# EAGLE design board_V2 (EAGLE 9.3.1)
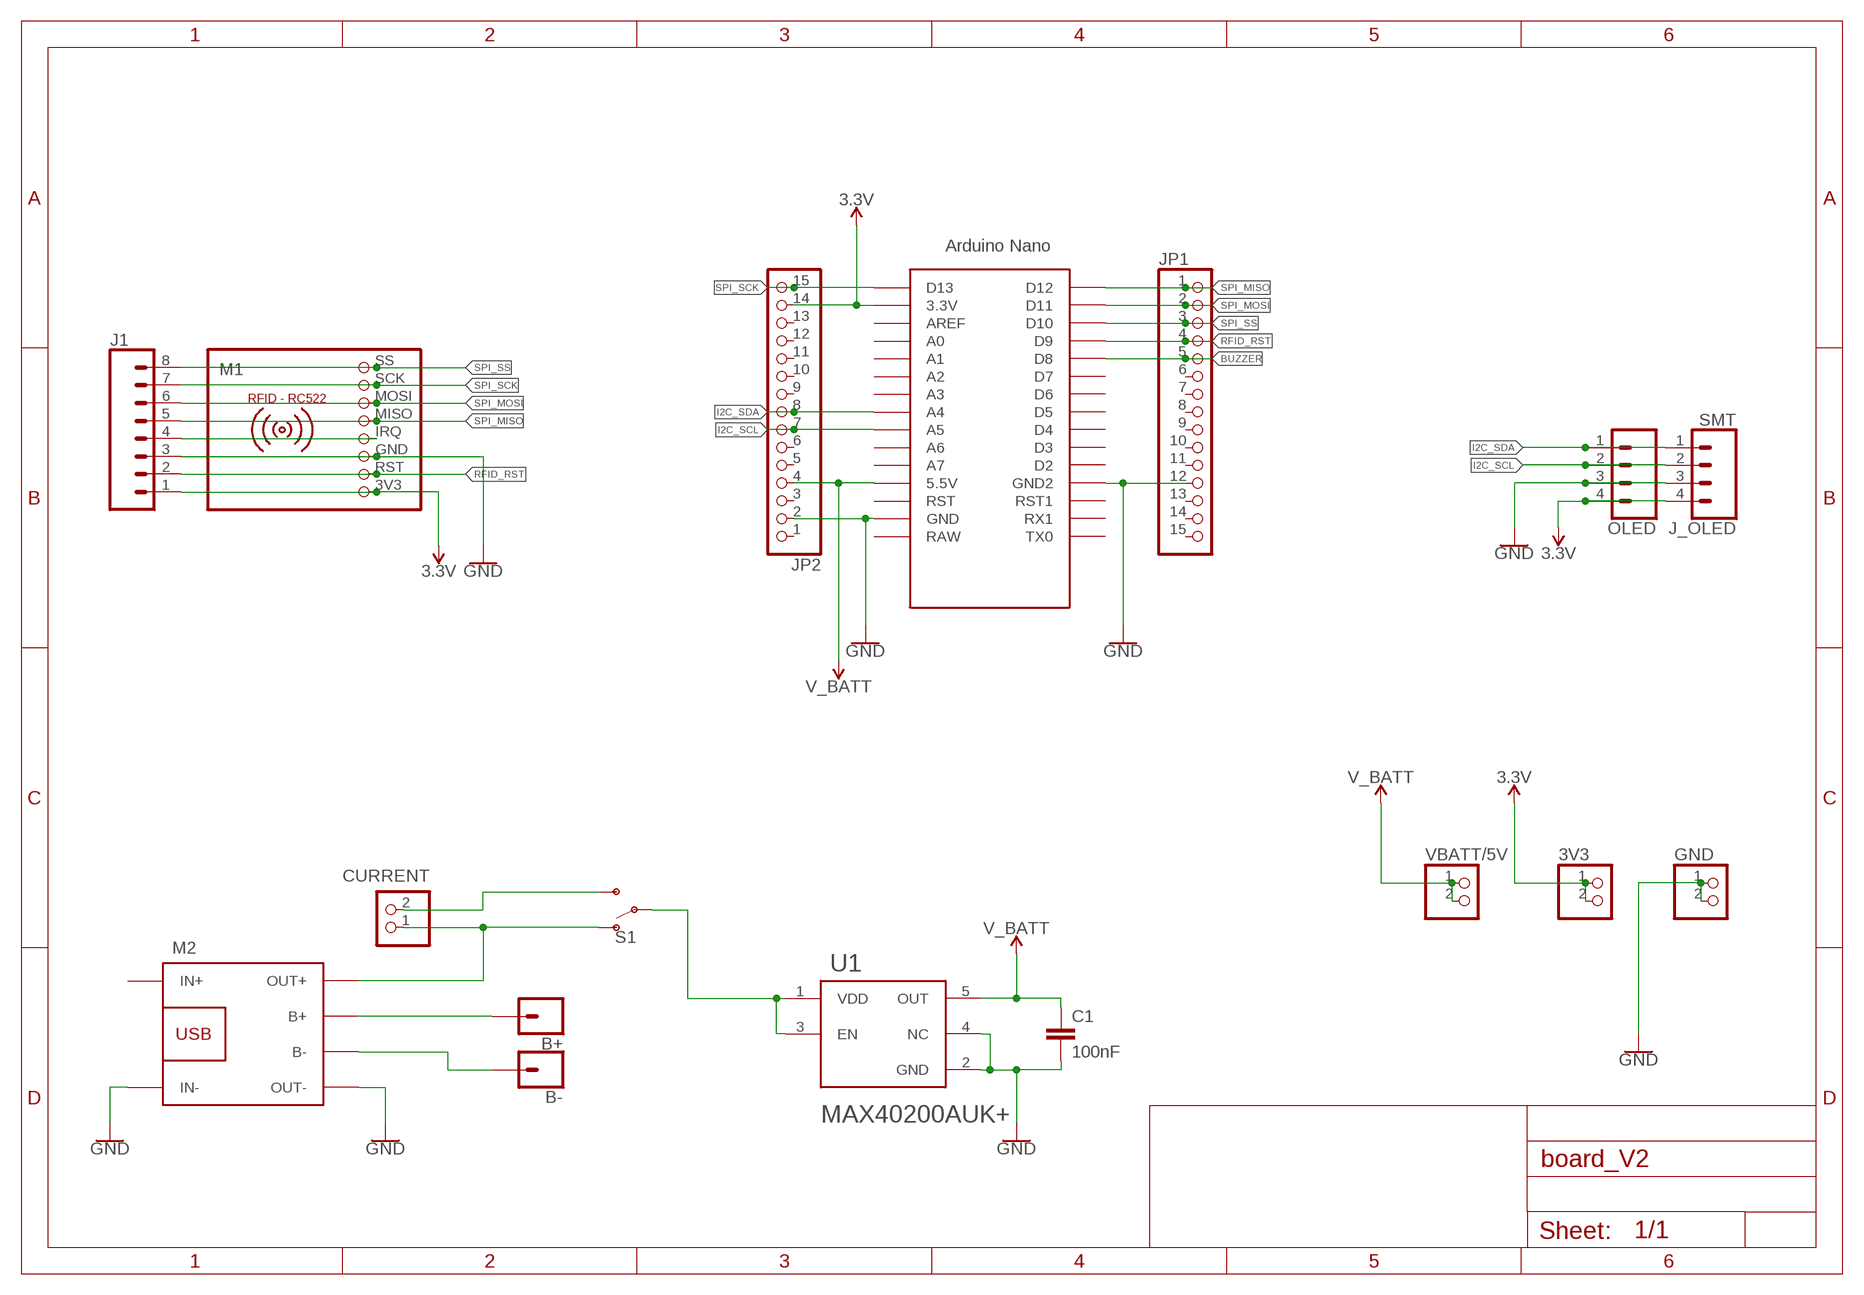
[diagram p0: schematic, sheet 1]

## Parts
3V3  PINHD-1X2  [1X02]
B+  CONN_01OFFSET  [1X01_OFFSET]
B-  CONN_01OFFSET  [1X01_OFFSET]
C1  100nF  C-EUC0805  [C0805]
CURRENT  PINHD-1X2  [1X02]
GND  PINHD-1X2  [1X02]
J1  CONN_08SMD-COMBO-FEMALE  [1X08_SMD_COMBINED]
J_OLED  SMT  CONN_04SMD_STRAIGHT_COMBO  [1X04_SMD_VERTICAL_COMBO]
JP1  PINHD-1X151X15_SMT  [1X15_SMT]
JP2  PINHD-1X151X15_SMT  [1X15_SMT]
M1  RFID-RC522  [RFID-RC522]
M2  BATTERY-CHARGER-LI-PROT  [BATTERY-CHARGER-LI-PROT]
OLED  CONN_04  [1X04]
S1  SWITCH-SPDT-PTH-11.6X4.0MM  [SWITCH_SPDT_PTH_11.6X4.0MM]
U1  MAXIM_ELECTRONICS_MAX40200AUK+MAXIM_ELECTRONICS_MAX40200AUK+_0_0  [MAXIM_ELECTRONICS_MAX40200AUK+_0]
U$1  NANO_ICSP-REMOVED  [NANO_ICSP-REMOVED]
VBATT/5V  PINHD-1X2  [1X02]

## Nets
3.3V [power]: 3V3.1 3V3.2 J1.1 J_OLED.4 JP2.14 M1.3V3 OLED.4 U$1.3.3V
BATT_VOUT [power]: S1.2(P) U1.1(VDD) U1.3(EN)
BUZZER: JP1.5 U$1.D8
GND [power]: C1.2 GND.1 GND.2 J1.3 J_OLED.3 JP1.12 JP2.2 M1.GND M2.IN- M2.OUT- OLED.3 U1.2(GND) U1.4(NC) U$1.GND U$1.GND1(GND2)
I2C_SCL: J_OLED.2 JP2.7 OLED.2 U$1.A5
I2C_SDA: J_OLED.1 JP2.8 OLED.1 U$1.A4
N$1 [power]: B+.1 M2.B+
N$2 [power]: CURRENT.1 M2.OUT+ S1.1(O)
N$3: J1.4 M1.IRQ
N$4 [power]: CURRENT.2 S1.3(S)
N$5 [power]: B-.1 M2.B-
RFID_RST: J1.2 JP1.4 M1.RST U$1.D9
SPI_MISO: J1.5 JP1.1 M1.MISO U$1.D12
SPI_MOSI: J1.6 JP1.2 M1.MOSI U$1.D11
SPI_SCK: J1.7 JP2.15 M1.SCK U$1.D13
SPI_SS: J1.8 JP1.3 M1.SS U$1.D10
V_BATT [power]: C1.1 JP2.4 U1.5(OUT) U$1.5V(5.5V) VBATT/5V.1 VBATT/5V.2
Unconnected: JP1.6 JP1.7 JP1.8 JP1.9 JP1.10 JP1.11 JP1.13 JP1.14 JP1.15 JP2.1 JP2.3 JP2.5 JP2.6 JP2.9 JP2.10 JP2.11 JP2.12 JP2.13 M2.IN+ U$1.A0 U$1.A1 U$1.A2 U$1.A3 U$1.A6 U$1.A7 U$1.AREF U$1.D2 U$1.D3 U$1.D4 U$1.D5 U$1.D6 U$1.D7 U$1.RAW U$1.RST U$1.RST1 U$1.RX1 U$1.TX0

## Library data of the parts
3V3 CURRENT GND VBATT/5V = pinhead:PINHD-1X2: PIN HEADER
B+ B- = SparkFun-Connectors:CONN_01: Single connection point. Often used as Generic Header-pin footprint for 0.1 inch spaced/style header connections
C1 = rcl:C-EU: CAPACITOR, European symbol; SPICEPREFIX: C
J1 = SparkFun-Connectors:CONN_08: Multi connection point. Often used as Generic Header-pin footprint for 0.1 inch spaced/style header connections On any of the 0.1 inch spaced packages, you can populate with these: Break Away Headers - Straight (PRT-00116) Break Away Male Headers - Right Angle (PRT-00553) Female Headers (PRT-00115)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; PROD_ID: CONN-10204; SF_ID: PRT-11543
J_OLED = SparkFun-Connectors:CONN_04: Multi connection point. Often used as Generic Header-pin footprint for 0.1 inch spaced/style header connections On any of the 0.1 inch spaced packages, you can populate with these: Break Away Headers - Straight (PRT-00116) Break Away Male Headers - Right Angle (PRT-00553) Female Headers (PRT-00115)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; PROD_ID: CONN-08511; VALUE: 1X04_SMD_STRAIGHT_COMBO
JP1 JP2 = pinhead+:PINHD-1X15: PIN HEADER
M1 = mfrc522-module:RFID-RC522: RFID-RC522 MFRC-522 based breakout board
M2 = diy-modules:BATTERY-CHARGER-LI-PROT: Lithium Battery 5V Charger with protection circuit More details available here: http://www.instructables.com/id/DIY-Lithium-ion-Battery-Charger/step4/TP4056-based-lithium-ion-battery-charger-module/ Click here to find device on ebay.com
OLED = SparkFun-Connectors:CONN_04: Multi connection point. Often used as Generic Header-pin footprint for 0.1 inch spaced/style header connections On any of the 0.1 inch spaced packages, you can populate with these: Break Away Headers - Straight (PRT-00116) Break Away Male Headers - Right Angle (PRT-00553) Female Headers (PRT-00115)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; PROD_ID: CONN-09696
S1 = SparkFun-Switches:SWITCH-SPDT: Single Pole, Double Throw (SPDT) Switch Single-pole, double-throw (SPDT) switch. Variant Overview SMD-AYZ0202 Surface Mount DPDT Switch (COM-00597) Used on e.g. LilyPad Arduino USB - ATmega32U4 Board PTH-11.6X4.0MM SPDT Mini Power Switch (COM-00102) Used on e.g. SparkFun Simon Says - Through-Hole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; PROD_ID: SWCH-08261; SF_SKU: COM-00102
U1 = Maxim Electronics - MAX40200AUK+:MAXIM_ELECTRONICS_MAX40200AUK+: IDEAL DIODE CURRENT SW, 5.5V, SOT23-5; CENTROID_NOT_SPECIFIED: No; DATASHEET: https://datasheets.maximintegrated.com/en/ds/MAX40200.pdf; DEVICE_CLASS_L1: Integrated Circuits (ICs); DEVICE_CLASS_L2: Power Management ICs; DEVICE_CLASS_L3: unset; DIGIKEY_DESCRIPTION: IC DIODE CURRENT SWITCH SOT23-5; DIGIKEY_PART_NUMBER: MAX40200AUK+-ND; FOOTPRINT_URL: https://pdfserv.maximintegrated.com/land_patterns/90-0174.PDF; HEIGHT: 1.45mm; LEAD_FREE: yes; MAX_JUNCTION_TEMP: +150°C; MAX_POWER_DISSIPATION: 312.6mW; MAX_SUPPLY_VOLTAGE: 5.5V; MF: Maxim Electronics; MFG_PACKAGE_IDENT: U5-1; MFG_PACKAGE_IDENT_DATE: 0; MFG_PACKAGE_IDENT_REV: J; MIN_SUPPLY_VOLTAGE: 1.5V; MOUSER_PART_NUMBER: 700-MAX40200AUK+; MPN: MAX40200AUK+; NOMINAL_SUPPLY_CURRENT: 7uA; NUMBER_OF_OUTPUTS: 1; OUTPUT_CURRENT: 1A; PACKAGE: SOT23-5; PREFIX: U; ROHS: yes; STANDOFF_HEIGHT: 0mm; TEMPERATURE_RANGE_HIGH: +125°C; TEMPERATURE_RANGE_LOW: -40°C; VERIFICATION_VERSION: 0.0.0.1
U$1 = Arduino-clone:NANO_ICSP-REMOVED

## Module BUZZER
Ports: 

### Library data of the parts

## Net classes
1 power: width 0.914 mm, clearance 0.254 mm

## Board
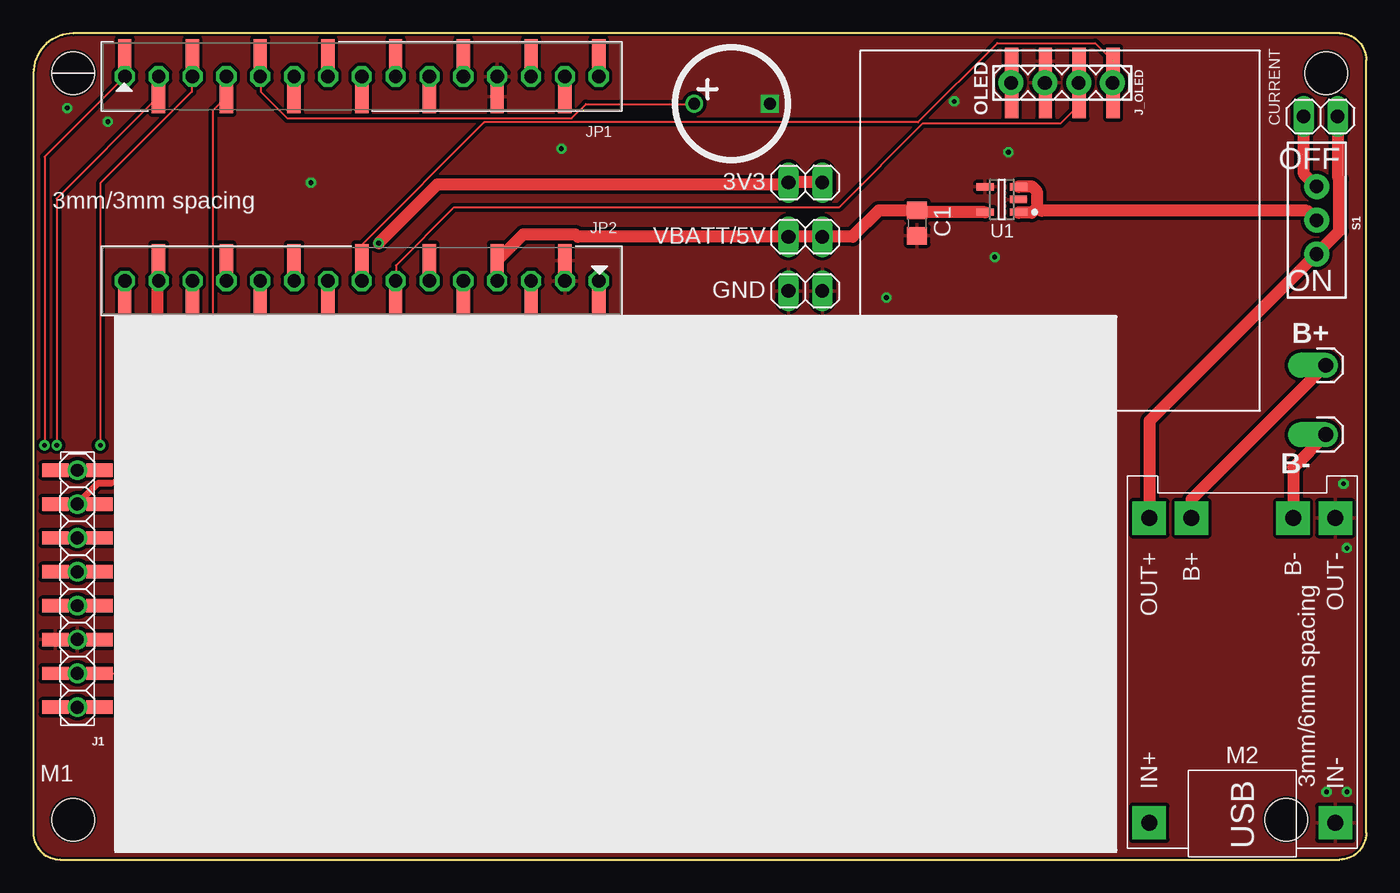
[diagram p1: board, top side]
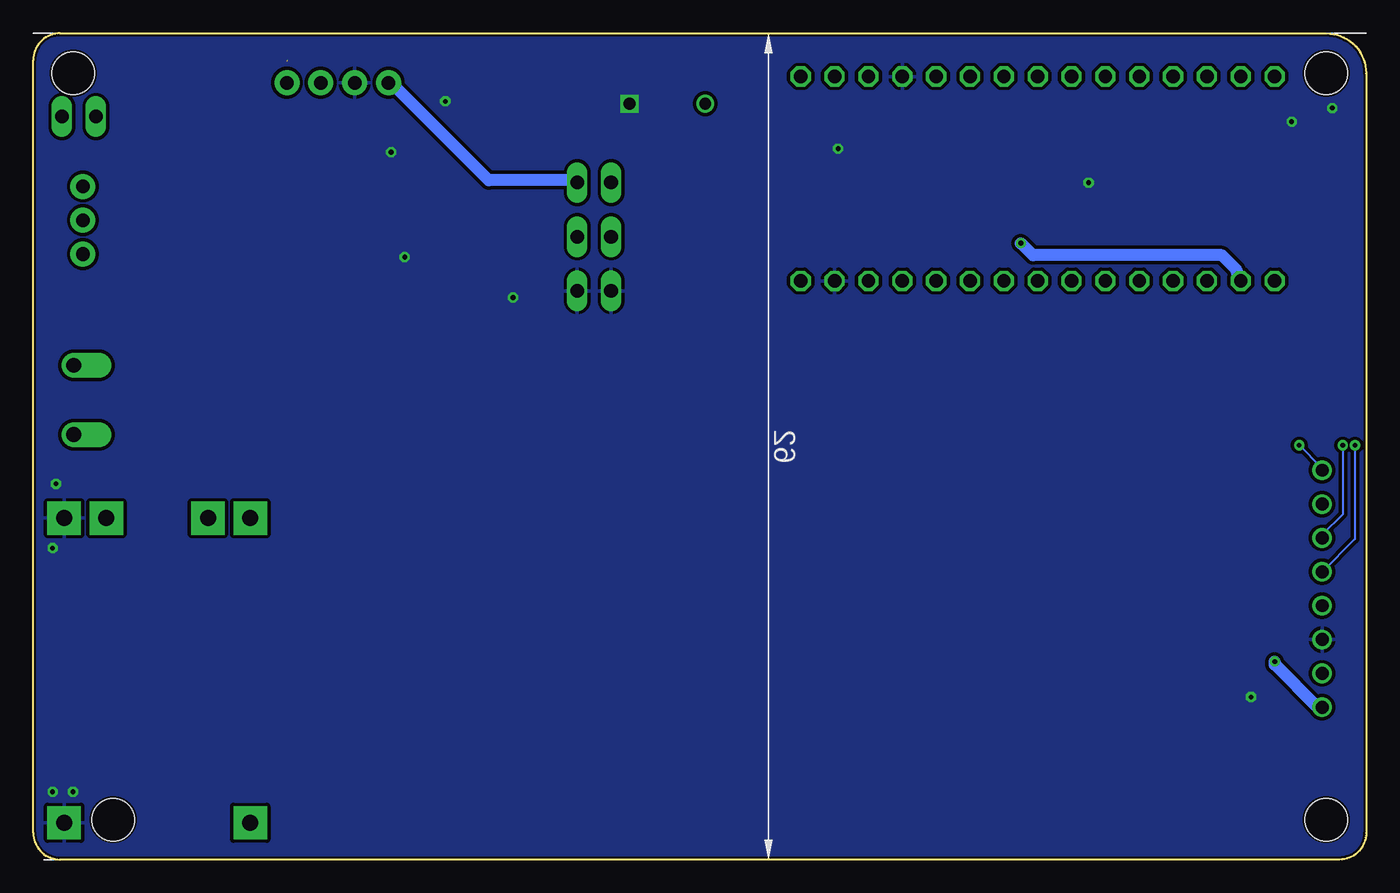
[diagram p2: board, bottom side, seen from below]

Size 100 x 62 mm. Coordinates in mm from the lower left corner, seen from the top.
Outline: 2,0 98,0 arc90 100,2 100,60 arc90 98,62 3,62 arc90 0,59 0,2 arc90 2,0
Copper layers (1*16): Top 0.035mm / dielectric 1.5mm / Bottom 0.035mm
Design rules "default *": minimum track width 6mil, minimum drill 0.35mm, track to track 6mil, track to pad 6mil, pad to pad 6mil, via to via 6mil, smd to smd 6mil, copper to edge 6mil, drill to drill 6mil, minimum pad ring 10mil, minimum via ring 8mil, stop-mask expansion 4mil, vias tented up to drill 0mil, thermal gap 10mil
Holes 3.2 mm at 3,59 3,3 94,3 97,59

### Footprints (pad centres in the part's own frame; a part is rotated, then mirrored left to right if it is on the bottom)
1X02 = drill 1.016 long: 1 -1.27,0; 2 1.27,0
1X01_OFFSET = drill 1.118 pad 1.88 offset: 1 0,0
C0805 = smd 1.3 x 1.5: 1 -0.95,0; 2 0.95,0
1X08_SMD_COMBINED = smd 1 x 2: 1 0,1.65; 1@2 0,-1.65; 2 2.54,-1.65; 2@2 2.54,1.65; 3 5.08,1.65; 3@2 5.08,-1.65; 4 7.62,-1.65; 4@2 7.62,1.65; 5 10.16,1.65; 5@2 10.16,-1.65; 6 12.7,-1.65; 6@2 12.7,1.65; 7 15.24,1.65; 7@2 15.24,-1.65; 8 17.78,-1.65; 8@2 17.78,1.65
1X04_SMD_VERTICAL_COMBO = smd 1 x 2: 1 0,-1.65; 1-2 0,1.65; 2 2.54,1.65; 2-2 2.54,-1.65; 3 5.08,-1.65; 3-2 5.08,1.65; 4 7.62,1.65; 4-2 7.62,-1.65
1X15_SMT = smd 1 x 2.5: 1 -17.78,1.52; 2 -15.24,-1.52; 3 -12.7,1.52; 4 -10.16,-1.52; 5 -7.62,1.52; 6 -5.08,-1.52; 7 -2.54,1.52; 8 0,-1.52; 9 2.54,1.52; 10 5.08,-1.52; 11 7.62,1.52; 12 10.16,-1.52; 13 12.7,1.52; 14 15.24,-1.52; 15 17.78,1.52
RFID-RC522 = drill 0.965: 3V3 -8.89,0; GND -3.81,0; IRQ -1.27,0; MISO 1.27,0; MOSI 3.81,0; RST -6.35,0; SCK 6.35,0; SS 8.89,0
BATTERY-CHARGER-LI-PROT = drill 1.2 pad 2.5 square: B+ 10.795,3.81; B- 10.795,-3.81; IN+ -12.065,6.985; IN- -12.065,-6.985; OUT+ 10.795,6.985; OUT- 10.795,-6.985
1X04 = drill 1.016 pad 1.88: 1 0,0; 2 2.54,0; 3 5.08,0; 4 7.62,0
SWITCH_SPDT_PTH_11.6X4.0MM = drill 1.016 pad 1.88: 1 0,2.54; 2 0,0; 3 0,-2.54
MAXIM_ELECTRONICS_MAX40200AUK+_0 = smd 1.3 x 0.55: 1 -1.25,0.95; 2 -1.25,0; 3 -1.25,-0.95; 4 1.25,-0.95; 5 1.25,0.95
NANO_ICSP-REMOVED = drill 1 octagon: 3.3V -10.16,24.13; 5V -10.16,-1.27; A0 -10.16,19.05; A1 -10.16,16.51; A2 -10.16,13.97; A3 -10.16,11.43; A4 -10.16,8.89; A5 -10.16,6.35; A6 -10.16,3.81; A7 -10.16,1.27; AREF -10.16,21.59; D2 5.182,1.27; D3 5.182,3.81; D4 5.182,6.35; D5 5.182,8.89; D6 5.182,11.43; D7 5.182,13.97; D8 5.182,16.51; D9 5.182,19.05; D10 5.182,21.59; D11 5.182,24.13; D12 5.182,26.67; D13 -10.16,26.67; GND -10.16,-6.35; GND1 5.182,-1.27; RAW -10.16,-8.89; RST -10.16,-3.81; RST1 5.182,-3.81; RX1 5.182,-6.35; TX0 5.182,-8.89

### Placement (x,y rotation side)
3V3  57.93,50.8 180 top
B+  96.96,37.09 90 top
B-  96.96,31.88 90 top
C1  66.31,47.75 270 top
CURRENT  96.58,55.75 180 top
GND  57.93,42.67 180 top
J1  3.3,11.43 90 top
J_OLED  81.01,58.27 180 top
JP1  24.64,58.77 0 top
JP2  24.64,43.43 180 top
M1  3.3,20.32 90 top
M2  90.7,14.82 90 top
OLED  80.97,58.29 180 top
S1  96.28,47.97 180 top
U1  72.66,49.53 180 top
U$1  33.53,53.58 90 top
VBATT/5V  57.93,46.74 180 top

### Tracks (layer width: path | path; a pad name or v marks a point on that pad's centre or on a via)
3.3V  (via drill 0.35)
  Top 0.914: 3V3.1 59.13,50.83 56.69,50.83 3V3.2 56.24,50.67 30.33,50.67 v25.91,46.25 | JP2.14 9.37,44.88 9.37,43.43 U$1.3.3V 9.3,42.98 9.3,33.3 7.87,31.88 7.87,15.88 v6.86,14.86 | M1.3V3 J1.1 | OLED.4 73.35,56.66 J_OLED.4
  Bottom 0.914: OLED.4 73.3,58.22 73.08,58.22 65.84,50.98 59.36,50.98 59.21,50.83 3V3.1 | M1.3V3 3.66,11.43 6.86,14.63 v6.86,14.86 | v25.91,46.25 24.99,45.34 10.82,45.34 9.75,44.27 9.75,44.2 9.68,44.12 9.68,43.97 9.45,43.74 9.45,43.43 U$1.3.3V
BATT_VOUT
  Top 0.914: 75.29,48.92 74.91,48.54 73.91,48.54 U1.1 | 75.29,48.92 75.29,50.14 74.91,50.52 73.91,50.52 U1.3 | 75.29,48.92 75.67,48.69 95.56,48.69 96.24,48.01 S1.2
BUZZER  (via drill 0.89)
  Top 0.152: v49.59,56.72 49.53,56.69 41.45,56.69 40.39,55.63 19.05,55.63 17.07,57.61 17.07,58.75 U$1.D8 16.99,58.83 16.99,60.27 JP1.5
GND  (via drill 0.35, 0.89)
  other vias: 55.26,56.72 39.62,53.34 5.59,55.37 2.54,56.39 8.64,12.19 98.55,5.08 97.03,5.08 98.55,23.37 98.3,28.19 72.14,45.21 64.01,42.16 73.15,53.09 69.09,56.9 20.83,50.8
  pour Top: -5.08,68.04 117.06,68.04 117.06,-5.08 -5.08,-5.08
  pour Bottom: -5.08,68.04 117.06,68.04 117.06,-5.08 -5.08,-5.08
I2C_SCL
  Top 0.152: JP2.7 27.2,41.91 27.2,43.36 U$1.A5 27.2,43.43 27.2,44.58 31.55,48.92 60.43,48.92 66.75,55.24 77.09,55.24 78.42,56.57 78.47,56.57
  Top 0.508: 78.47,56.57 78.43,56.61 OLED.2 78.43,56.66 J_OLED.2
I2C_SDA  (1 unrouted)
  Top 0.152: U$1.A4 24.61,43.43 24.61,44.88 JP2.8 24.69,44.96 24.69,46.18 33.83,55.32 66.37,55.32 72.31,61.27 79.67,61.27 80.96,59.98 81.01,59.98 | OLED.1 81.01,58.33 J_OLED.1
N$1
  Top 0.914: B+.1 86.89,27.02 M2.B+
N$2
  Top 0.914: CURRENT.1 97.92,55.7 97.92,51.13 97.99,51.05 97.99,47.17 96.32,45.49 S1.1 95.94,45.11 83.74,32.92 83.74,25.68 M2.OUT+
N$3
  Top 0.914: M1.IRQ J1.4
N$4
  Top 0.914: CURRENT.2 95.33,55.7 95.33,51.44 96.24,50.52 S1.3
N$5
  Top 0.914: B-.1 94.51,29.43 M2.B-
RFID_RST
  Top 0.152: U$1.D9 JP1.4 14.48,57.23 13.49,56.24 13.49,20.34 7.11,13.97 5.08,13.97
  Top 0.508: 5.08,13.97 M1.RST J1.2
SPI_MISO  (via drill 0.35)
  Top 0.152: JP1.1 6.86,58.83 U$1.D12 0.84,52.73 v0.84,31.09
  Top 0.914: M1.MISO J1.5
  Bottom 0.152: M1.MISO 0.84,24.05 v0.84,31.09
SPI_MOSI  (via drill 0.35)
  Top 0.152: U$1.D11 9.37,58.75 9.37,57.3 JP1.2 9.37,57.23 1.75,49.61 v1.75,31.09
  Top 0.914: M1.MOSI J1.6
  Bottom 0.152: v1.75,31.09 1.75,25.91 3.28,24.38 3.28,24.16 M1.MOSI
SPI_SCK
  Top 0.152: U$1.D13 6.86,43.36 JP2.15 6.86,29.29 5.81,28.25
  Top 0.508: J1.7 M1.SCK 4.88,28.25 5.81,28.25
SPI_SS  (via drill 0.35)
  Top 0.152: JP1.3 11.96,60.27 11.96,58.83 U$1.D10 11.89,58.75 11.89,57.61 5.03,50.75 v5.03,31.09
  Top 0.508: J1.8 M1.SS
  Bottom 0.152: v5.03,31.09 3.35,29.41 3.35,29.26 M1.SS
V_BATT
  Top 0.914: U1.5 66.43,48.58 C1.1 63.43,48.7 61.47,46.74 VBATT/5V.1 VBATT/5V.2 40.84,46.74 40.67,46.91 36.76,46.91 JP2.4 U$1.5V

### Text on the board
tPlace: OFF | 3mm/3mm spacing | ON | 3mm/6mm spacing

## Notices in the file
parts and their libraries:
SparkFun-Connectors: Licensing: Creative Commons ShareAlike 4.0 International - https://creativecommons.org/licenses/by-sa/4.0
diy-modules: Released under the Creative Commons Attribution 4.0 International License: http://creativecommons.org/licenses/by/4.0
